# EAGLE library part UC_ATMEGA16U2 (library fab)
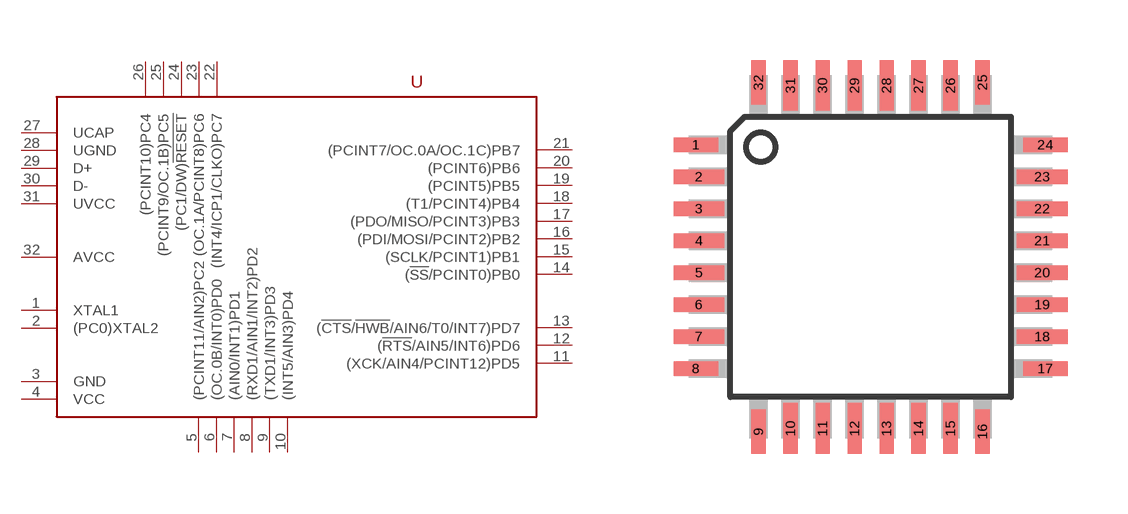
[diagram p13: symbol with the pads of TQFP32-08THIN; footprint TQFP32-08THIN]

Designator prefix -

## UC_ATMEGA16U2-TQ  [TQFP32-08THIN]
1  XTAL1
2  (PC0)XTAL2
3  GND
4  VCC
5  (PCINT11/AIN2)PC2
6  (OC.0B/INT0)PD0
7  (AIN0/INT1)PD1
8  (RXD1/AIN1/INT2)PD2
9  (TXD1/INT3)PD3
10  (INT5/AIN3)PD4
11  (XCK/AIN4/PCINT12)PD5
12  (!RTS!/AIN5/INT6)PD6
13  (!CTS!/!HWB!/AIN6/T0/INT7)PD7
14  (!SS!/PCINT0)PB0
15  (SCLK/PCINT1)PB1
16  (PDI/MOSI/PCINT2)PB2
17  (PDO/MISO/PCINT3)PB3
18  (T1/PCINT4)PB4
19  (PCINT5)PB5
20  (PCINT6)PB6
21  (PCINT7/OC.0A/OC.1C)PB7
22  (INT4/ICP1/CLKO)PC7
23  (OC.1A/PCINT8)PC6
24  (PC1/DW)!RESET
25  (PCINT9/OC.1B)PC5
26  (PCINT10)PC4
27  UCAP
28  UGND
29  D+
30  D-
31  UVCC
32  AVCC

## Footprint TQFP32-08THIN (pad centres in mm)
smd 1.118 x 0.356: 1 -4.369,2.8; 8 -4.369,-2.8; 17 4.369,-2.8; 24 4.369,2.8
smd 1.27 x 0.356: 2 -4.293,2; 3 -4.293,1.2; 4 -4.293,0.4; 5 -4.293,-0.4; 6 -4.293,-1.2; 7 -4.293,-2; 18 4.293,-2; 19 4.293,-1.2; 20 4.293,-0.4; 21 4.293,0.4; 22 4.293,1.2; 23 4.293,2
smd 0.356 x 1.118: 9 -2.8,-4.369; 16 2.8,-4.369; 25 2.8,4.369; 32 -2.8,4.369
smd 0.356 x 1.27: 10 -2,-4.293; 14 1.2,-4.293; 15 2,-4.293; 26 2,4.293; 27 1.2,4.293; 31 -2,4.293
smd 0.35 x 1.27: 11 -1.2,-4.293; 12 -0.4,-4.293; 13 0.4,-4.293; 28 0.4,4.293; 29 -0.4,4.293; 30 -1.2,4.293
